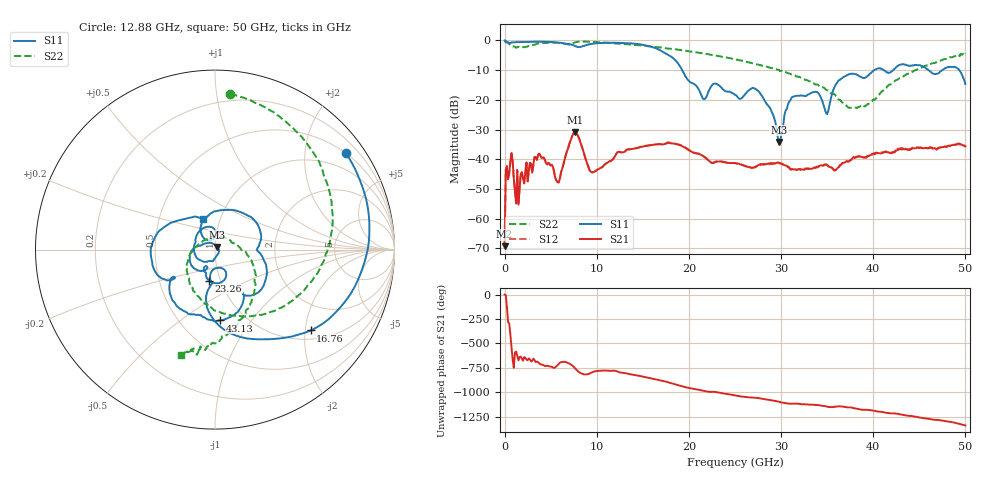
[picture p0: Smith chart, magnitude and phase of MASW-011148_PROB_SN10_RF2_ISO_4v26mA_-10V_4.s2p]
!Keysight Technologies,N5247A,US51170177,A.10.64.09
!Date: Saturday, May 29, 2021 13:17:48
!Correction: S11(Full 2 Port(1,2))
!S21(Full 2 Port(1,2))
!S12(Full 2 Port(1,2))
!S22(Full 2 Port(1,2))
!S2P File: Measurements: S11, S21, S12, S22:
# Hz S  dB  R 50
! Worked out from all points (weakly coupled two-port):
!   401 points, 10 MHz to 50 GHz, reference 50 ohm
!   highest |S21| = -30.93 dB at 7.633 GHz (marker M1); lowest = -69.3 dB at 10 MHz (marker M2)
!   lowest |S11| = -34.2 dB at 29.75 GHz (marker M3), VSWR 1.04, Z = 51.2 + j1.55 ohm
!   |S11| at or under -10 dB: 19.28 GHz to 40.11 GHz (20.83 GHz wide, 70.2 % of centre); 41.14 GHz to 42.17 GHz (1.032 GHz wide, 2.48 % of centre); 45.99 GHz to 47.48 GHz (1.489 GHz wide, 3.19 % of centre)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
!   |S22| runs from -22.8 to 0.0 dB; largest |S21 - S12| = 0.001
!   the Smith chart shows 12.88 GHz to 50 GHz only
!   S11 on the Smith chart (normalised r, x): 12.88 GHz: 0.50, +2.97; 16.76 GHz: 1.22, -2.14; 23.26 GHz: 0.88, -0.32; 43.13 GHz: 0.77, -0.72; 50 GHz: 0.83, +0.29
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1e7  -0.01 -1.8  -69.26 1.9  -68.21 -73.8  -0.02 -1.0
3.84925e8  -0.62 -51.6  -46.75 80.1  -46.80 81.1  -0.88 -32.9
8.84825e8  -0.64 -97.5  -40.60 52.5  -40.63 52.7  -1.99 -61.2
2.384525e9  -0.53 -163.9  -41.13 53.6  -41.12 54.0  -2.12 -116.7
5.75885e9  -0.69 131.0  -47.70 -4.1  -47.73 -4.2  -0.85 171.1
7.633475e9  -1.84 104.6  -30.93 -33.7  -30.94 -33.7  -0.67 151.2
8.383325e9  -2.07 102.3  -35.69 -89.0  -35.68 -89.1  -0.41 138.9
9.5081e9  -1.13 88.9  -44.48 -75.5  -44.40 -75.6  -0.52 123.6
1.288242e10  -0.87 36.3  -37.65 -81.7  -37.63 -81.4  -1.20 84.4
1.675665e10  -3.12 -40.2  -34.94 -155.7  -34.87 -155.5  -2.32 43.1
2.163068e10  -19.75 -83.4  -39.12 92.6  -39.01 92.3  -4.43 -7.9
2.325535e10  -15.08 -100.6  -40.79 76.9  -40.63 76.6  -5.27 -25.0
2.5005e10  -18.28 -120.4  -41.27 48.7  -41.26 47.8  -6.36 -43.7
2.75045e10  -16.94 -168.4  -42.03 21.3  -42.23 21.7  -8.15 -70.9
2.975405e10  -34.22 51.0  -41.16 -18.0  -41.16 -18.3  -9.86 -96.8
3.112878e10  -19.34 -150.4  -43.32 -37.7  -43.55 -36.4  -11.49 -112.9
3.337832e10  -17.53 135.6  -43.17 -48.3  -43.28 -48.6  -14.11 -143.2
3.5003e10  -24.81 113.6  -41.94 -67.5  -41.89 -67.1  -16.76 -167.1
3.762748e10  -11.22 33.4  -40.10 -76.4  -40.26 -76.7  -22.70 119.7
4.175165e10  -10.94 -57.5  -37.87 -133.9  -37.78 -132.3  -14.88 -8.9
4.312638e10  -8.06 -86.0  -36.72 -150.6  -36.15 -151.4  -12.39 -26.1
5e10  -14.68 111.5  -35.62 99.4  -35.92 100.1  -4.22 -108.2
